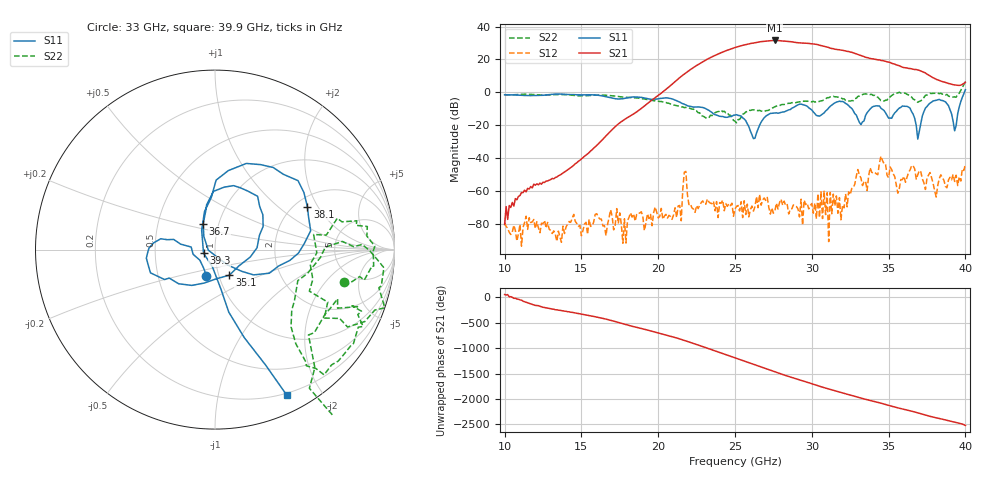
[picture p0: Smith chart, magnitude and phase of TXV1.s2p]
!Keysight Technologies,M9808A,MY58100618,A.14.70.03
!Date: Monday, February 27, 2023 13:18:40
!Correction: S11(C  2-Port  )
!S21(C  2-Port  )
!S12(C  2-Port  )
!S22(C  2-Port  )
!S2P File: Measurements: S11, S21, S12, S22:
# Hz S  RI  R 50
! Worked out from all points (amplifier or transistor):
!   301 points, 10 GHz to 40 GHz, reference 50 ohm
!   highest |S21| = 31.5 dB at 27.6 GHz (marker M1)
!   |S21| within 3 dB of that: 25.49 GHz to 30.55 GHz (5.066 GHz wide, 18.1 % of centre)
!   unconditionally stable (mu >= 1): start of sweep to 35.69 GHz; 35.71 GHz to 39.63 GHz
!   at 15 GHz: K = 158706.79, MAG = -31.6 dB, |S12| = -87.5 dB
!   at 25 GHz: K = 74.20, MAG = 27.5 dB, |S12| = -71.2 dB
!   at 40 GHz: K = 60.41, MSG = 24.9 dB, |S12| = -43.7 dB
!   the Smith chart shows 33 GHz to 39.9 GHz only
!   S11 on the Smith chart (normalised r, x): 33 GHz: 0.87, -0.26; 35.1 GHz: 1.12, -0.33; 36.7 GHz: 0.84, +0.25; 38.1 GHz: 2.32, +1.63; 39.3 GHz: 0.88, -0.04; 39.9 GHz: 0.18, -1.59
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1e10  0.7122 0.4442  4.91e-05 7.92e-05  1.32e-06 -0.000104  0.0798 0.8219
1.5e10  0.6462 -0.5172  0.00796 0.00492  1.35e-05 4.01e-05  0.7546 0.177
2e10  -0.1945 -0.5969  0.7399 0.3  -0.000117 -9.16e-05  0.2019 -0.4918
2.34e10  -0.2461 -0.0788  5.764 9.794  -0.000415 3.4e-05  -0.1624 -0.1152
2.42e10  -0.1785 0.0388  15.18 -6.976  -0.000208 0.000474  -0.2113 -0.143
2.5e10  -0.1421 0.1428  -7.694 -21.68  0.000215 -0.000173  -0.1293 -0.0213
2.58e10  -0.0665 0.0867  -28.07 7.536  -8.58e-05 -0.000379  -0.1924 0.1724
2.65e10  0.0741 -0.0107  -0.7053 33.43  0.00025 0.000169  -0.2075 0.1795
2.76e10  0.1984 -0.1252  33.91 -16.57  0.000211 0.000131  0.0184 0.3614
2.82e10  0.1252 -0.2181  1.163 -36.14  0.000443 0.000184  0.088 0.4134
2.89e10  0.0452 -0.3626  -30.29 -13.31  -0.00033 1.24e-05  0.1998 0.4302
3e10  0.0862 -0.2737  -5.361 29.51  -0.000214 -0.000345  0.2587 0.4391
3.1e10  -0.2451 -0.1608  23.52 2.179  -0.000839 0.000213  0.6154 0.2914
3.2e10  -0.2247 -0.4738  3.584 -18.64  0.000341 0.000131  0.5372 0.3276
3.3e10  -0.0478 -0.1454  -13.8 -3.106  0.00412 0.00155  0.7198 -0.1808
3.5e10  0.00811 -0.1624  6.805 4.748  -0.00238 0.000765  0.6283 -0.2927
3.51e10  0.0801 -0.1425  7.187 3.574  0.00401 -0.00346  0.6091 -0.3812
3.67e10  -0.0656 0.1451  -0.6007 -4.879  -0.00459 0.000117  0.5866 -0.0449
3.81e10  0.515 0.2385  -2.115 1.282  0.000484 0.000423  0.761 -0.5295
3.93e10  -0.0638 -0.02  0.7638 1.482  0.00024 -0.0019  0.5538 -0.4623
3.99e10  0.3993 -0.8103  1.8 0.4063  0.00206 -0.00357  0.98 -1.391
4e10  0.5601 -1.06  2.009 -0.0768  0.0036 0.00549  1.113 -1.805
